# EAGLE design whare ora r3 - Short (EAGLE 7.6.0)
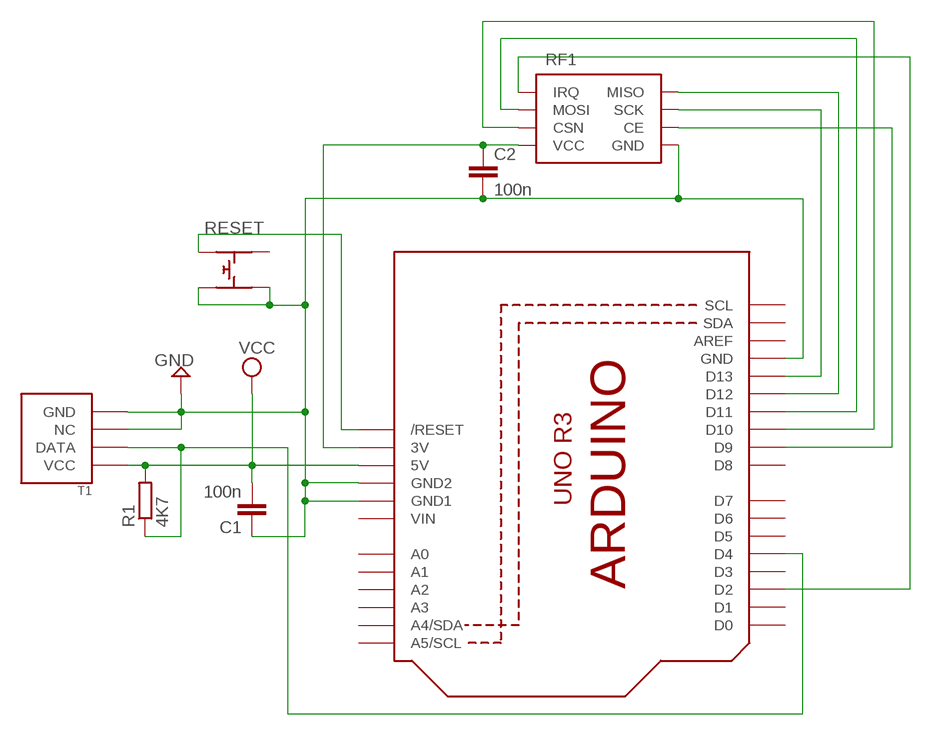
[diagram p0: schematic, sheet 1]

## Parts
C1  100n  C-EUC0805  [C0805]
C2  100n  C-EUC0805  [C0805]
Q1  ARDUINOR3-NOIOREFSHORT  [ARDUINOR3-NOTEXT-SHORT]
R1  4K7  R-EU_M0805  [M0805]
RESET  SPST  [FSM-SMT]
RF1  NRF24L01+RF2  [RF2]
T1  DHT22  [DHT22]

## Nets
CE: Q1.D9 RF1.P$3(CE)
CS: Q1.D10 RF1.P$4(CSN)
GND: C1.1 C2.2 Q1.GND Q1.GND1 Q1.GND2 RESET.P$3 RESET.P$4 RF1.P$1(GND) T1.P$3(NC) T1.P$4(GND)
IRQ: Q1.D2 RF1.P$8(IRQ)
MISO: Q1.D12 RF1.P$7(MISO)
MOSI: Q1.D11 RF1.P$6(MOSI)
N$1: Q1.RESET(/RESET) RESET.P$1
N$2: Q1.D4 R1.1 T1.P$2(DATA)
SCK: Q1.D13 RF1.P$5(SCK)
VCC: C1.2 Q1.5V R1.2 T1.P$1(VCC)
VDD: C2.1 Q1.3V RF1.P$2(VCC)
Unconnected: Q1.A0 Q1.A1 Q1.A2 Q1.A3 Q1.A4(A4/SDA) Q1.A5(A5/SCL) Q1.AREF Q1.D0 Q1.D1 Q1.D3 Q1.D5 Q1.D6 Q1.D7 Q1.D8 Q1.SCL Q1.SDA RESET.P$2

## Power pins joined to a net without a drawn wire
VIN: Q1.VIN

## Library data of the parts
C1 C2 = rcl:C-EU: CAPACITOR, European symbol
Q1 = adafruit:ARDUINOR3-NOIOREF
R1 = rcl:R-EU_: RESISTOR, European symbol
RESET = Callum:SPST
RF1 = Callum:NRF24L01+
T1 = Callum:DHT

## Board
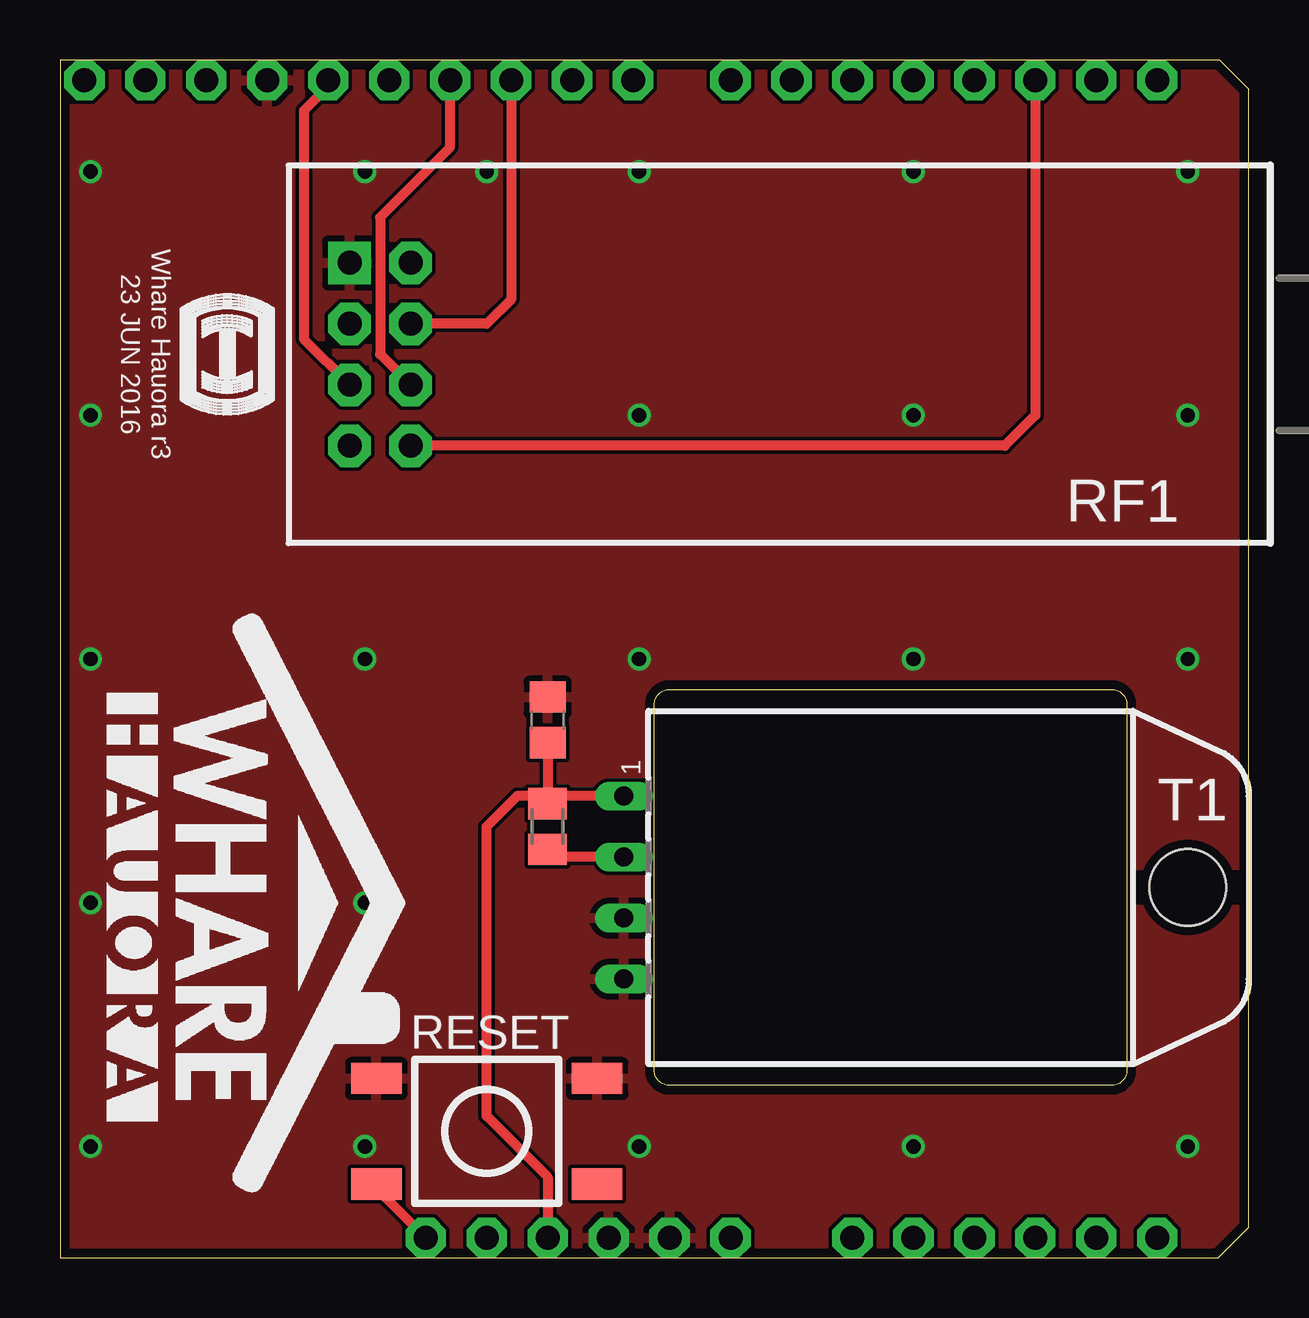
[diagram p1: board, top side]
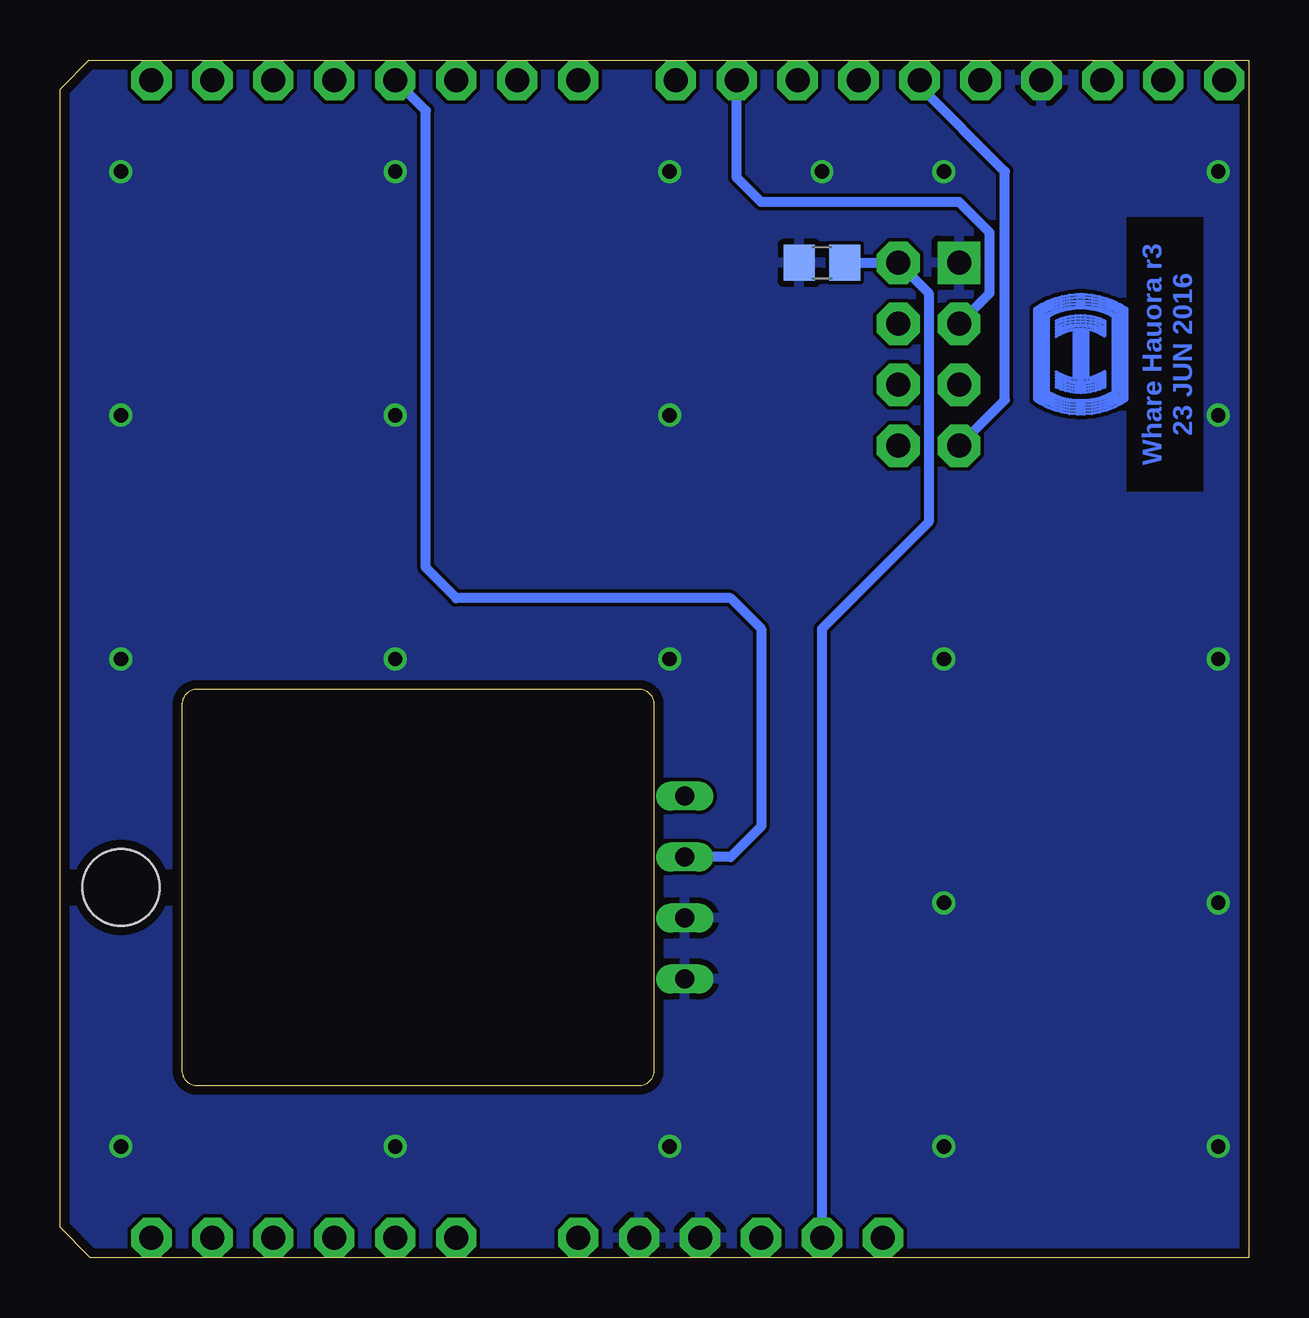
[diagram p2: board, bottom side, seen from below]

Size 49.53 x 49.91 mm. Coordinates in mm from the lower left corner, seen from the top.
Outline: 25.4,23.69 43.81,23.69 arc-90 44.45,23.05 44.45,7.81 arc-90 43.81,7.18 25.4,7.18 arc-90 24.77,7.81 24.77,23.05 arc-90 25.4,23.69
Copper layers (1*16): Top 0.0356mm / dielectric 1.5011mm / Bottom 0.0356mm
Design rules "OSHpark DRC *": minimum track width 6mil, minimum drill 13mil, track to track 6mil, track to pad 6mil, pad to pad 6mil, via to via 6mil, smd to smd 6mil, copper to edge 15mil, drill to drill 6mil, minimum pad ring 7mil, minimum via ring 7mil, stop-mask expansion 3mil, vias tented up to drill 30mil, thermal gap 10mil
bRestrict: area 1.9,31.9 to 5.1,43.4

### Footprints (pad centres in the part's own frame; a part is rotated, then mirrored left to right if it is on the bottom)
C0805 = smd 1.3 x 1.5: 1 -0.95,0; 2 0.95,0
ARDUINOR3-NOTEXT-SHORT = drill 1 pad 1.676 octagon: 3V 19.05,2.54; 5V 21.59,2.54; A0 34.29,2.54; A1 36.83,2.54; A2 39.37,2.54; A3 41.91,2.54; A4 44.45,2.54; A5 46.99,2.54; AREF 7.366,50.8; D0 46.99,50.8; D1 44.45,50.8; D2 41.91,50.8; D3 39.37,50.8; D4 36.83,50.8; D5 34.29,50.8; D6 31.75,50.8; D7 29.21,50.8; D8 25.146,50.8; D9 22.606,50.8; D10 20.066,50.8; D11 17.526,50.8; D12 14.986,50.8; D13 12.446,50.8; GND 9.906,50.8; GND1 26.67,2.54; GND2 24.13,2.54; RESET 16.51,2.54; SCL 2.286,50.8; SDA 4.826,50.8; VIN 29.21,2.54
M0805 = smd 1.3 x 1.6: 1 -0.95,0; 2 0.95,0
FSM-SMT = smd 1.3 x 2.1: P$1 -2.2,4.6; P$2 -2.2,-4.6; P$3 2.2,4.6; P$4 2.2,-4.6
RF2 = drill 1 pad 1.778 square: P$1 0,0 | drill 1 pad 1.778 octagon: P$2 -2.54,0; P$3 0,2.54; P$4 -2.54,2.54; P$5 0,5.08; P$6 -2.54,5.08; P$7 0,7.62; P$8 -2.54,7.62
DHT22 = drill 0.8 long: P$1 0,0; P$2 2.54,0; P$3 5.08,0; P$4 7.62,0 | hole 3.2: 3.81,23.495

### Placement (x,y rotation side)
C1  20.32,22.42 270 top
C2  17.78,41.47 180 bottom
Q1  -1.27,-1.71 0 top
R1  20.32,17.97 90 top
RESET  17.78,5.27 90 top
RF1  12.07,41.47 180 top
T1  23.5,19.24 270 top
U$1  [MY-LOGO-COPPER]  6.99,37.66 270 bottom
U$2  [MY-LOGO-SMALL]  6.99,37.66 270 top
U$3  [WHAREHAUORA]  2.16,26.23 270 top

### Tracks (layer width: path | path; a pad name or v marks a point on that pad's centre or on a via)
CE
  Bottom 0.406: RF1.P$3 10.79,40.2 10.79,42.74 12.07,44.01 20.32,44.01 21.34,45.02 Q1.D9
CS
  Top 0.406: RF1.P$4 17.78,38.93 18.8,39.94 Q1.D10
GND  (via drill 0.6)
  other vias: 24.13,35.12 1.27,45.28 24.13,4.64 1.27,24.96 1.27,4.64 12.7,45.28 35.56,35.12 46.99,24.96 35.56,45.28 24.13,45.28 46.99,35.12 12.7,4.64 24.13,24.96 35.56,4.64 35.56,24.96 12.7,14.8 46.99,45.28 12.7,24.96 1.27,35.12 1.27,14.8 46.99,4.64 17.78,45.28
  pour Bottom: 0,0.19 48.26,0.19 49.53,1.46 49.53,48.45 48.26,49.72 0,49.72
  pour Top: 0,49.72 48.26,49.72 49.53,48.45 49.53,1.46 48.26,0.19 0,0.19
IRQ
  Top 0.406: Q1.D2 40.64,35.12 39.37,33.85 RF1.P$8
MISO
  Bottom 0.406: RF1.P$7 10.16,35.75 10.16,45.28 13.72,48.83 Q1.D12
MOSI
  Top 0.406: RF1.P$6 13.34,37.66 13.34,43.37 16.26,46.29 Q1.D11
N$1
  Top 0.406: RESET.P$1 13.18,2.89 Q1.RESET
N$2
  Top 0.406: T1.P$2 20.64,16.7 R1.1
  Bottom 0.406: Q1.D4 34.29,47.82 34.29,28.77 33.02,27.5 21.59,27.5 20.32,26.23 20.32,17.97 21.59,16.7 T1.P$2
SCK
  Top 0.406: RF1.P$5 10.16,38.29 10.16,47.82 11.18,48.83 Q1.D13
VCC
  Top 0.406: T1.P$1 20.32,19.24 | 20.32,19.24 19.05,19.24 17.78,17.97 17.78,5.91 20.32,3.37 Q1.5V | 20.32,19.24 R1.2 C1.2
VDD
  Bottom 0.406: C2.1 RF1.P$2 13.34,40.2 13.34,30.67 17.78,26.23 Q1.3V

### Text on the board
Bottom: 23 JUN 2016 | Whare Hauora r3
tPlace: 23 JUN 2016 | Whare Hauora r3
